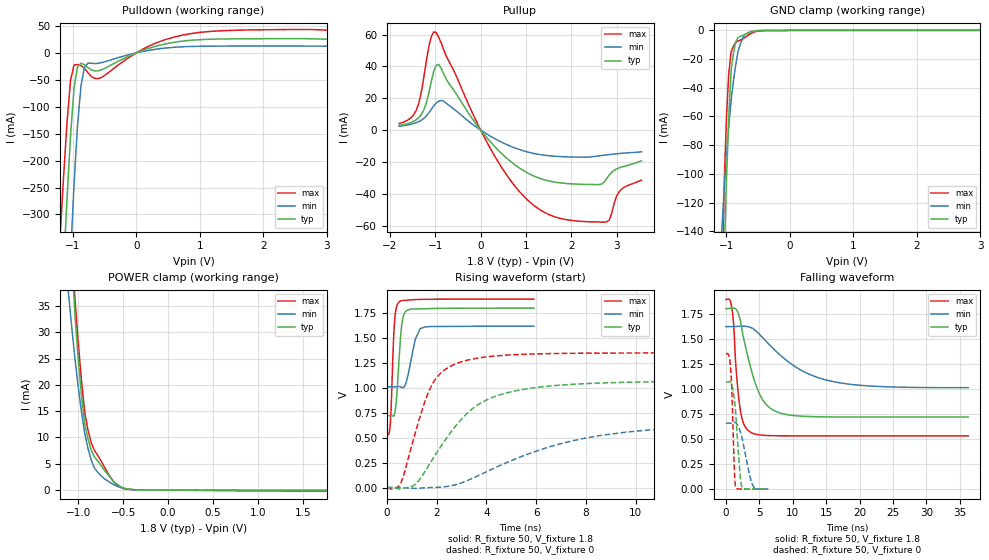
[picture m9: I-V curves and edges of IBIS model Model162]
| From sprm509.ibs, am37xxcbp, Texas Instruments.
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| Model based on original model for DSIPHY_WIO_ADDON_GPIOWRAPPER
|   Sub model FBPB_HS00L10_PU1_1P8
[model]   Model162
|[Input Load]   PU
|[Output Drive] SC00LB10
|Voltage   1.8V
|Mode   I/O
Model_type   I/O
Polarity   Non-Inverting
Enable   Active-Low
Vinl =  0.63
Vinh =  1.17
Cref =  15pF
Rref =  100.0000M
Vref =  0V
Vmeas =  0.9
C_comp   1.429432p   1.270657p   1.602015p
[Model Spec]
Vinl   0.63   0.567   0.6615
Vinh   1.17   1.053   1.2285
[Temperature Range]   25   125   -40
[Voltage Range]   1.8   1.62   1.89
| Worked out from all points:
|   slope of the pulldown table from 0 to 0.27 V, typ, clamps not added: 24.3 ohm
|   slope of the pullup table from 0 to 0.27 V, typ, clamps not added: 29.7 ohm
|   GND clamp passes 1 mA (typ) near -0.60 V on its own axis
|   POWER clamp passes 1 mA (typ) near -0.56 V on its own axis
|   rising waveform, R_fixture 50, V_fixture 1.8: 20-80 % time 176ps typ, 309ps min, 124ps max; typ from 0.72 V to 1.8 V
|   rising waveform, R_fixture 50, V_fixture 0: 20-80 % time 2.17ns typ, 4.91ns min, 1.1ns max; typ from 0.001 V to 1.07 V
|   falling waveform, R_fixture 50, V_fixture 1.8: 20-80 % time 2.71ns typ, 7.23ns min, 940ps max; typ from 1.8 V to 0.72 V
|   falling waveform, R_fixture 50, V_fixture 0: 20-80 % time 703ps typ, 1.22ns min, 396ps max; typ from 1.07 V to 0.002 V
[POWER_clamp]
-1.8V     362.5mA    191.4mA    412.8mA
-1.109V   56.76mA    37.74mA    60.51mA
-1.073V   44.67mA    31.25mA    47.93mA
-1.036V   33.52mA    25.07mA    36.72mA
-1V       25.06mA    19.75mA    28.2mA
-963.6mV  18.11mA    14.99mA    20.91mA
-927.3mV  12.67mA    10.8mA     14.87mA
-890.9mV  9.734mA    7.935mA    11.44mA
-818.2mV  6.293mA    4.153mA    7.536mA
-636.4mV  2.249mA    1.342mA    2.34mA
-418.2mV  128.7uA    129.3uA    104.4uA
1.764V    -96.73uA   -46.48uA   -163.5uA
[Pulldown]
-1.8V     -1.718A    -2.61A     -1.406A
-1.2V     -527.4mA   -844.5mA   -339.9mA
-1.145V   -396mA     -683.1mA   -229.1mA
-1.091V   -269mA     -526.7mA   -127.5mA
-1.036V   -153.6mA   -378.9mA   -51.17mA
-981.8mV  -66.33mA   -245.6mA   -22.67mA
-927.3mV  -26mA      -136.2mA   -21.54mA
-872.7mV  -19.34mA   -61.98mA   -23.69mA
-763.6mV  -27.2mA    -19.05mA   -36.72mA
-545.5mV  -31.39mA   -18.17mA   -45.46mA
872.7mV   23.46mA    11.88mA    35.92mA
3.545V    25.34mA    12.51mA    41.58mA
[Pullup]
-1.8V     2.903mA    2.423mA    4.112mA
-1.418V   6.595mA    4.711mA    12.64mA
-1.255V   12.69mA    7.42mA     33.24mA
-1.091V   30.4mA     13mA       58.69mA
-981.8mV  40.63mA    17.02mA    61.3mA
-818.2mV  35.38mA    18.12mA    50.59mA
272.7mV   -9.179mA   -4.728mA   -14.55mA
1.255V    -29.75mA   -15.09mA   -48.97mA
2.564V    -34.17mA   -16.31mA   -57.57mA
2.782V    -30.25mA   -15.5mA    -57.49mA
3.055V    -23.63mA   -14.68mA   -38.61mA
3.545V    -19.25mA   -13.56mA   -31.41mA
[GND_clamp]
-1.8V     -2.82A     -1.192A    -3.165A
-1.073V   -235.8mA   -138.4mA   -192.1mA
-1.036V   -159.6mA   -110.8mA   -107.6mA
-1V       -103.8mA   -87.86mA   -60.73mA
-963.6mV  -60.04mA   -67.29mA   -29.86mA
-927.3mV  -28.26mA   -49.09mA   -14.98mA
-890.9mV  -15.95mA   -35.49mA   -11.09mA
-854.5mV  -8.198mA   -24.09mA   -8.559mA
-818.2mV  -4.99mA    -14.87mA   -7.387mA
-709.1mV  -2.858mA   -3.093mA   -5.012mA
-527.3mV  -395.6uA   -260.4uA   -751.2uA
3.6V      0A         0A         0A
[Ramp]
dV/dt_f  0.6509226/2.709959n   0.3680569/7.291109n   0.8172077/0.9364704n
dV/dt_r  0.6501752/2.174059n   0.400272/4.957263n   0.8213739/1.102497n
R_load = 50
[Rising Waveform]
R_fixture = 50
V_fixture = 1.8
V_fixture_min = 1.62
V_fixture_max = 1.89
0s        720.1mV    1.01V      534.4mV
144ps     721.2mV    1.011V     674.7mV
270ps     717.6mV    1.01V      1.516V
324ps     761.3mV    1.01V      1.717V
513ps     1.386V     1.012V     1.866V
594ps     1.631V     1.004V     1.874V
711ps     1.752V     1.018V     1.877V
1.143ns   1.791V     1.488V     1.885V
1.341ns   1.792V     1.595V     1.886V
5.913ns   1.799V     1.618V     1.89V
[Rising Waveform]
R_fixture = 50
V_fixture = 0
V_fixture_min = 0
V_fixture_max = 0
0s        1.173mV    1.024mV    -1.872mV
558ps     -12.81mV   1.262mV    44.86mV
1.197ns   46.33mV    -8.217mV   598.9mV
1.917ns   317.1mV    1.784mV    1.075V
2.574ns   557.3mV    18.15mV    1.219V
3.618ns   823.7mV    113.7mV    1.297V
5.022ns   961.9mV    272.9mV    1.331V
6.975ns   1.027V     439mV      1.345V
10.63ns   1.06V      579.7mV    1.35V
32.01ns   1.069V     657.1mV    1.35V
[Falling Waveform]
R_fixture = 50
V_fixture = 1.8
V_fixture_min = 1.62
V_fixture_max = 1.89
0s        1.8V       1.62V      1.89V
612ps     1.802V     1.62V      1.883V
963ps     1.805V     1.62V      1.773V
1.575ns   1.788V     1.622V     1.157V
2.259ns   1.645V     1.624V     749.1mV
3.753ns   1.199V     1.61V      566.4mV
5.886ns   855.1mV    1.484V     536.8mV
8.613ns   751.1mV    1.308V     532.9mV
16.8ns    720.6mV    1.063V     532.6mV
36.26ns   720mV      1.012V     532.6mV
[Falling Waveform]
R_fixture = 50
V_fixture = 0
V_fixture_min = 0
V_fixture_max = 0
0s        1.069V     658.8mV    1.35V
450ps     1.073V     658.7mV    1.327V
756ps     1.059V     659mV      1.165V
909ps     1.033V     660.6mV    949mV
1.251ns   908.3mV    666mV      221.3mV
1.494ns   728.2mV    660.6mV    12.46mV
2.106ns   160.9mV    585.6mV    2.877mV
2.412ns   19.4mV     511.7mV    2.362mV
4.023ns   2.104mV    39.03mV    1.866mV
6.345ns   1.596mV    2.593mV    1.787mV
